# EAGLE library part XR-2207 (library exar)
VOLTAGE CONTROLLED OSCILLATOR
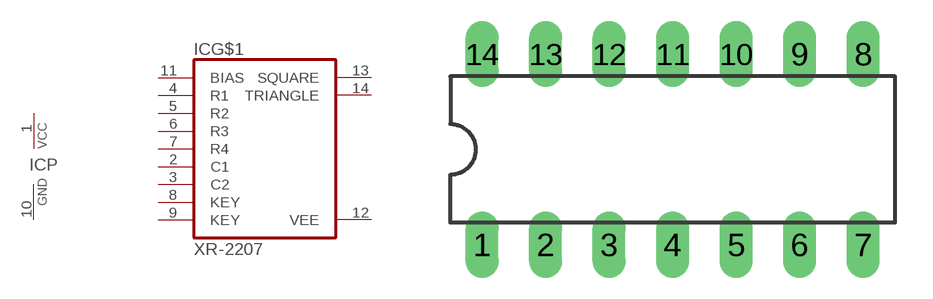
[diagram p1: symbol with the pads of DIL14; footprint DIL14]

Designator prefix IC; gates G$1=XR-2207 P=PWRN

## XR-2207 (OC_FARNELL: unknown; OC_NEWARK: unknown)  [DIL14]
1  P:VCC  pwr
2  G$1:C1  in
3  G$1:C2  in
4  G$1:R1  in
5  G$1:R2  in
6  G$1:R3  in
7  G$1:R4  in
8  G$1:KEY  in
9  G$1:KEY  in
10  P:GND  pwr
11  G$1:BIAS  in
12  G$1:VEE  pwr
13  G$1:SQUARE  out
14  G$1:TRIANGLE  out

## Footprint DIL14 (pad centres in mm)
Dual In Line Package
drill 0.813 long: 1 -7.62,-3.81; 2 -5.08,-3.81; 3 -2.54,-3.81; 4 0,-3.81; 5 2.54,-3.81; 6 5.08,-3.81; 7 7.62,-3.81; 8 7.62,3.81; 9 5.08,3.81; 10 2.54,3.81; 11 0,3.81; 12 -2.54,3.81; 13 -5.08,3.81; 14 -7.62,3.81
